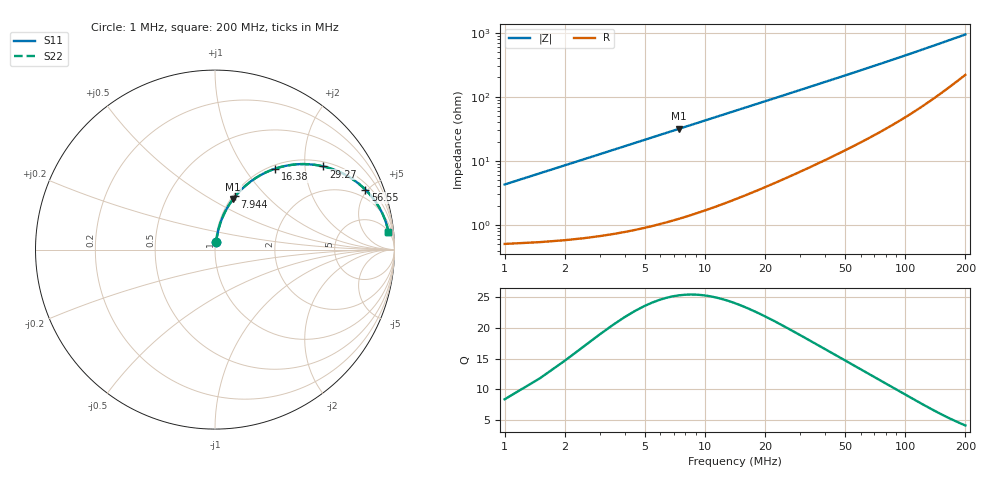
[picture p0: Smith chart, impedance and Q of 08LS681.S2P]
! Coilcraft 0805LS-681 Chip Inductor
! 18 September 2002
# MHZ S MA R 50
!Freq  MagS11  AngS11  MagS21  AngS21  MagS12  AngS12  MagS22  AngS22
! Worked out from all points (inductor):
!   403 points, 1 MHz to 200 MHz, reference 50 ohm
!   read as one part in series: L = 677 nH near 1.992 MHz
!   highest Q = 25.3 at 7.448 MHz (marker M1), where L = 677 nH
!   S11 on the Smith chart (normalised r, x): 1 MHz: 1.01, +0.09; 7.944 MHz: 1.03, +0.68; 16.38 MHz: 1.06, +1.39; 29.27 MHz: 1.13, +2.49; 56.55 MHz: 1.35, +4.85; 200 MHz: 5, +18
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1  0.04258 80.8  0.9941 -2.4  0.9941 -2.4  0.04258 80.8
1.496  0.06339 81.5  0.9926 -3.6  0.9926 -3.6  0.06339 81.5
2.488  0.1048 80.6  0.9884 -6.0  0.9884 -6.0  0.1048 80.6
2.984  0.1252 79.8  0.9855 -7.2  0.9855 -7.2  0.1252 79.8
3.976  0.1656 77.8  0.9786 -9.5  0.9786 -9.5  0.1656 77.8
5.464  0.2245 74.7  0.9652 -13.0  0.9652 -13.0  0.2245 74.7
7.448  0.2988 70.4  0.9426 -17.4  0.9426 -17.4  0.2988 70.4
7.944  0.3165 69.3  0.9362 -18.4  0.9362 -18.4  0.3165 69.3
9.432  0.3675 66.2  0.9156 -21.5  0.9156 -21.5  0.3675 66.2
11.416  0.4303 62.2  0.8856 -25.5  0.8856 -25.5  0.4303 62.2
13.896  0.5001 57.6  0.8455 -30.0  0.8455 -30.0  0.5001 57.6
16.376  0.5607 53.5  0.8042 -34.1  0.8042 -34.1  0.5607 53.5
21.832  0.6656 45.6  0.7156 -41.7  0.7156 -41.7  0.6656 45.6
29.272  0.7613 37.5  0.6096 -49.5  0.6096 -49.5  0.7613 37.5
34.232  0.8046 33.3  0.5503 -53.4  0.5503 -53.4  0.8046 33.3
44.152  0.8617 27.0  0.4556 -59.3  0.4556 -59.3  0.8617 27.0
56.552  0.9022 21.7  0.3707 -64.1  0.3707 -64.1  0.9022 21.7
67.464  0.9234 18.4  0.3165 -67.0  0.3165 -67.0  0.9234 18.4
100.696  0.9535 12.3  0.2148 -71.4  0.2148 -71.4  0.9535 12.3
133.928  0.9644 9.1  0.1598 -72.6  0.1598 -72.6  0.9644 9.1
167.16  0.9689 7.1  0.1259 -72.2  0.1259 -72.2  0.9689 7.1
200  0.9707 5.8  0.1035 -70.7  0.1035 -70.7  0.9707 5.8
